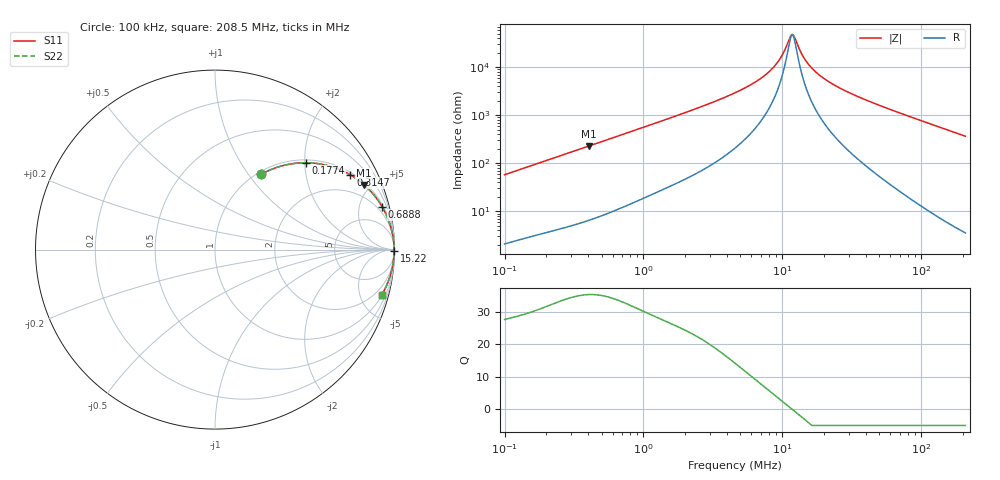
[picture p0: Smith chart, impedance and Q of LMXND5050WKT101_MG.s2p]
! LMXND5050WKT101_MG  S-PARAMETER MODEL  ( General Type )
! Model Generated by TAIYO YUDEN Corporation (https://www.yuden.co.jp/en/)
! Version 1.0
! TAIYO YUDEN Control No. 191023NI43SB-FBB
! Copyright(c) 2019 TAIYO YUDEN CO.,LTD. All Rights Reserved.
! Product Description (link to TY-COMPAS)
! https://ds.yuden.co.jp/TYCOMPAS/or/detail?pn=LMXND5050WKT101MMG&u=M
! Products Name : Inductors
! Characteristics :
!  Inductance : 100 uH , SRF(min) : 7.0 MHz , DC Resistance(max) : 1.02 Ohm
!  Rated Current : Saturation :420 mA , Temp Rise : 400 mA (40 degC)
!  Case Size : 4.9 x 4.9 / 0.193 x 0.193 [mm/inch] , Thickness : 2 / 0.079 [mm/inch]
!  (Conditions: Temperature = 25 degC , DC Bias Current/Voltage = 0A / 0V)
! External Node Assignments :
!  1  o---GGG---o  2
! GND o---------o GND
! Frequency Range : 0.1MHz  -  208.503118MHz  [ 402 STEP ]
# MHz S RI R 50
! Freq[MHz].  S11 Real  S11 Imag  S21 Real  S21 Imag  S12 Real  S12 Imag  S22 Real  S22 Imag
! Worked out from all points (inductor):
!   401 points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, 100 kHz to 208.5 MHz, reference 50 ohm
!   read as one part in series: L = 91.4 uH near 103.9 kHz
!   highest Q = 35.2 at 403.4 kHz (marker M1), where L = 89.9 uH
!   self-resonance near 11.65 MHz
!   S11 on the Smith chart (normalised r, x): 100 kHz: 1.04, +1.15; 177.4 kHz: 1.07, +2.03; 314.7 kHz: 1.10, +3.56; 688.8 kHz: 1.23, +7.75; 15.22 MHz: open; 208.5 MHz: 1.07, -7.33
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0.1  0.2578 0.4197  0.7422 -0.4197  0.7422 -0.4197  0.2578 0.4197
0.177392  0.5066 0.4839  0.4934 -0.4839  0.4934 -0.4839  0.5066 0.4839
0.314678  0.7544 0.4162  0.2456 -0.4162  0.2456 -0.4162  0.7544 0.4162
0.359709  0.7988 0.3869  0.2012 -0.3869  0.2012 -0.3869  0.7988 0.3869
0.403402  0.8317 0.3602  0.1683 -0.3602  0.1683 -0.3602  0.8317 0.3602
0.688773  0.9313 0.2383  0.0687 -0.2383  0.0687 -0.2383  0.9313 0.2383
1.293906  0.9768 0.1336  0.0232 -0.1336  0.0232 -0.1336  0.9768 0.1336
2.778523  0.9933 0.0612  0.00673 -0.0612  0.00673 -0.0612  0.9933 0.0612
4.654297  0.9965 0.0329  0.00347 -0.0329  0.00347 -0.0329  0.9965 0.0329
6.564688  0.9974 0.0191  0.00257 -0.0191  0.00257 -0.0191  0.9974 0.0191
8.415604  0.9978 0.0106  0.00224 -0.0106  0.00224 -0.0106  0.9978 0.0106
9.80545  0.9979 0.00576  0.00213 -0.00576  0.00213 -0.00576  0.9979 0.00576
11.20862  0.9979 0.0016  0.00208 -0.0016  0.00208 -0.0016  0.9979 0.0016
11.64522  0.9979 0.000421  0.00207 -0.000421  0.00207 -0.000421  0.9979 0.000421
12.33221  0.9979 -0.00135  0.00206 0.00135  0.00206 0.00135  0.9979 -0.00135
13.83017  0.9979 -0.00491  0.00208 0.00491  0.00208 0.00491  0.9979 -0.00491
15.21656  0.9979 -0.00792  0.00211 0.00792  0.00211 0.00792  0.9979 -0.00792
16.42508  0.9979 -0.0104  0.00215 0.0104  0.00215 0.0104  0.9979 -0.0104
19.88316  0.9977 -0.0168  0.00231 0.0168  0.00231 0.0168  0.9977 -0.0168
25.98091  0.9972 -0.0269  0.00275 0.0269  0.00275 0.0269  0.9972 -0.0269
59.08252  0.9925 -0.0738  0.00754 0.0738  0.00754 0.0738  0.9925 -0.0738
208.5031  0.9286 -0.2527  0.0714 0.2527  0.0714 0.2527  0.9286 -0.2527
